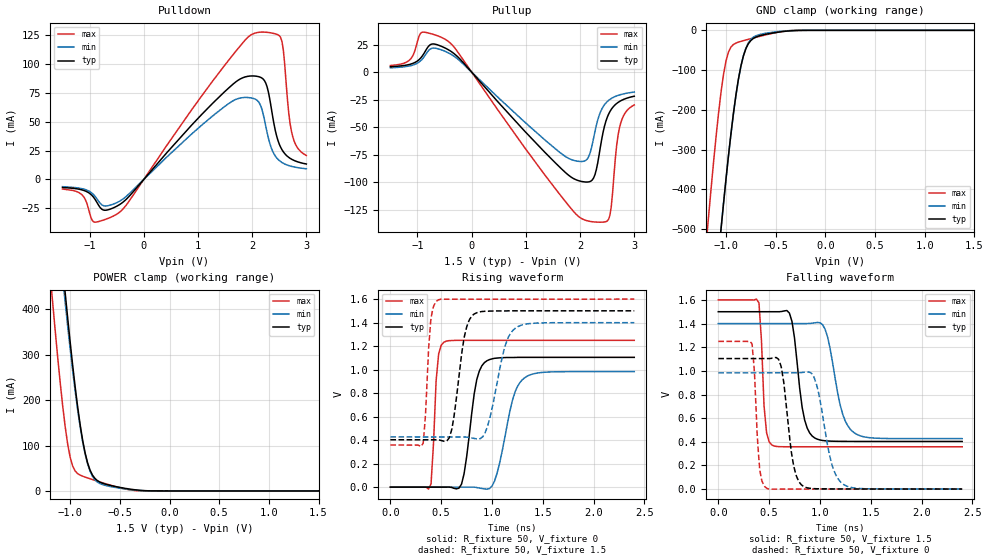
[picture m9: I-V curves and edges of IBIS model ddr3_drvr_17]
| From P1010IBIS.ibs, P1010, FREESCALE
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| * 8520 DDR3 Driver Model - 17 Ohm Setting *
[Model]   ddr3_drvr_17
Model_type I/O
Polarity   Non-Inverting
Vinl = 0.575V
Vinh = 0.925V
Vmeas = 0.75V
Cref = 0
Rref = 50
Vref = 0.75V
|   typ   min   max
C_comp   3.648430e-12   2.038680e-12   4.817870e-12
[Receiver Thresholds]
Vth   =  0.750V
Vinh_ac  =  0.175V
Vinh_dc  =  0.100V
Vinl_ac  = -0.175V
Vinl_dc  = -0.100V
|   typ   min   max
[Voltage range]   1.5V   1.4V   1.6V
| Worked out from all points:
|   slope of the pulldown table from 0 to 0.225 V, typ, clamps not added: 18.3 ohm
|   slope of the pullup table from 0 to 0.225 V, typ, clamps not added: 18 ohm
|   GND clamp passes 1 mA (typ) near -0.33 V on its own axis
|   POWER clamp passes 1 mA (typ) near -0.28 V on its own axis
|   falling waveform, R_fixture 50, V_fixture 1.5: 20-80 % time 91.6ps typ, 133ps min, 43.5ps max; typ from 1.5 V to 0.403 V
|   rising waveform, R_fixture 50, V_fixture 0: 20-80 % time 99.4ps typ, 146ps min, 44.5ps max; typ from 0 V to 1.1 V
|   falling waveform, R_fixture 50, V_fixture 0: 20-80 % time 89.7ps typ, 128ps min, 45.2ps max; typ from 1.1 V to 0.001 V
|   rising waveform, R_fixture 50, V_fixture 1.5: 20-80 % time 98.5ps typ, 143ps min, 46.5ps max; typ from 0.403 V to 1.5 V
[Pulldown]
| Warnings regarding non-monotonicity are expected
| Voltage   I(typ)   I(min)   I(max)
-1.5V     -6.943mA   -6.27mA    -8.283mA
-1.125V   -9.276mA   -8.191mA   -14.06mA
-925mV    -15.52mA   -13.22mA   -36.74mA
-750mV    -26.41mA   -22.64mA   -35.27mA
-450mV    -21.89mA   -18.94mA   -28.47mA
1.575V    79.47mA    65.9mA     103.7mA
2.125V    88.85mA    66.72mA    127.3mA
2.275V    80.21mA    40.73mA    127.3mA
2.525V    27.91mA    15.44mA    122.9mA
2.575V    23.89mA    13.96mA    112.1mA
2.725V    17.56mA    11.32mA    41.68mA
3V        13.34mA    9.202mA    20.75mA
[GND_clamp]
| Voltage   I(typ)   I(min)   I(max)
-1.5V     -1.83A     -1.803A    -1.463A
-1.2V     -918.5mA   -909.4mA   -538.8mA
-1.175V   -846mA     -838.3mA   -467.5mA
-1.05V    -500.5mA   -498.8mA   -155.7mA
-1V       -374.3mA   -374.5mA   -77.03mA
-925mV    -208.7mA   -210.1mA   -35.53mA
-875mV    -123mA     -123.8mA   -29.71mA
-825mV    -64.79mA   -64.04mA   -26.02mA
-775mV    -33.87mA   -31.49mA   -22.62mA
-675mV    -14.65mA   -11.59mA   -16.08mA
-300mV    -558.2uA   -260.8uA   -231.8uA
1.5V      1.426uA    9.416uA    7.097nA
[Pullup]
| Warnings regarding non-monotonicity are expected
| Voltage   I(typ)   I(min)   I(max)
-1.5V     4.946mA    3.957mA    6.022mA
-1.125V   7.341mA    5.906mA    12.1mA
-925mV    13.8mA     11.15mA    36.06mA
-750mV    25.28mA    21.42mA    34.91mA
-425mV    20.2mA     17.42mA    27.68mA
1.725V    -90.86mA   -76.41mA   -117.1mA
2.2V      -98.86mA   -70.77mA   -135.6mA
2.35V     -75.39mA   -39.55mA   -136.2mA
2.525V    -38.24mA   -25.66mA   -133.7mA
2.575V    -33.81mA   -23.91mA   -122.3mA
2.725V    -26.69mA   -20.71mA   -51mA
3V        -21.81mA   -18.04mA   -29.75mA
[POWER_clamp]
| Warnings about POWER_clamp data never reaching
| zero are expected, and this is okay as long as
| the 0V data are around 10uA or less
| Voltage   I(typ)   I(min)   I(max)
-1.5V     1.587A     1.494A     1.288A
-1.2V     797.2mA    753.3mA    475mA
-1.175V   734.5mA    694.6mA    412.6mA
-1.1V     552mA      523.4mA    238.4mA
-1.05V    436.4mA    415mA      141.5mA
-1V       328.1mA    313.2mA    74.16mA
-925mV    186.2mA    179.4mA    38.2mA
-825mV    62.3mA     59.8mA     28.63mA
-775mV    34.82mA    32mA       25mA
-675mV    17.02mA    14mA       18mA
-300mV    1.425mA    937.9uA    241uA
1.5V      0A         0A         0A
|   typ   min   max
[Ramp]
dV/dt_r   0.66242/9.74685E-11   0.589801/1.44544E-10   0.74934/3.84995E-11
dV/dt_f   0.658119/9.00708E-11   0.583749/1.32332E-10   0.745099/3.75614E-11
[Falling Waveform]
R_fixture = 50
V_fixture = 1.5
V_fixture_min = 1.4
V_fixture_max = 1.6
| Time   V(typ)   V(min)   V(max)
0s        1.5V       1.4V       1.6V
400ps     1.5V       1.4V       1.575V
450ps     1.5V       1.4V       704.9mV
525ps     1.5V       1.4V       374.3mV
700ps     1.488V     1.4V       358.4mV
850ps     583.8mV    1.4V       358.4mV
950ps     432.1mV    1.406V     358.3mV
1.05ns    409mV      1.354V     358.3mV
1.325ns   403.6mV    484.6mV    358.3mV
2.4ns     403.1mV    427.1mV    358.3mV
[Rising Waveform]
R_fixture = 50
V_fixture = 0
V_fixture_min = 0
V_fixture_max = 0
| Time   V(typ)   V(min)   V(max)
0s        37.05uV    20.71uV    106.5nV
400ps     40.27uV    27uV       26.62mV
450ps     43.13uV    25.23uV    905.9mV
525ps     32.64uV    25.46uV    1.232V
700ps     25.44mV    17.82uV    1.249V
850ps     914.8mV    -3.331mV   1.249V
950ps     1.075V     -17.34mV   1.249V
1.225ns   1.103V     805.4mV    1.249V
1.325ns   1.104V     932.8mV    1.249V
2.4ns     1.104V     983mV      1.249V
[Falling Waveform]
R_fixture = 50
V_fixture = 0
V_fixture_min = 0
V_fixture_max = 0
| Time   V(typ)   V(min)   V(max)
0s        1.104V     983mV      1.249V
332.4ps   1.104V     982.5mV    1.226V
405.7ps   1.104V     982.6mV    184.7mV
479ps     1.104V     982.6mV    6.049mV
615.8ps   1.044V     982.6mV    603uV
738ps     215.1mV    982.6mV    744.1uV
835.8ps   24.63mV    987.3mV    743.6uV
958ps     3.609mV    907.7mV    743.6uV
1.217ns   1.129mV    49.37mV    743.6uV
2.4ns     1.023mV    1.338mV    743.6uV
[Rising Waveform]
R_fixture = 50
V_fixture = 1.5
V_fixture_min = 1.4
V_fixture_max = 1.6
| Time   V(typ)   V(min)   V(max)
0s        403.1mV    427.1mV    358.1mV
322.6ps   403.3mV    427mV      373.6mV
395.9ps   403.3mV    427mV      1.405V
469.2ps   402.3mV    427mV      1.592V
596.3ps   467.3mV    427mV      1.599V
728.3ps   1.282V     427mV      1.599V
826ps     1.474V     413.8mV    1.599V
938.4ps   1.496V     476.5mV    1.599V
1.241ns   1.5V       1.359V     1.599V
2.4ns     1.5V       1.399V     1.6V
